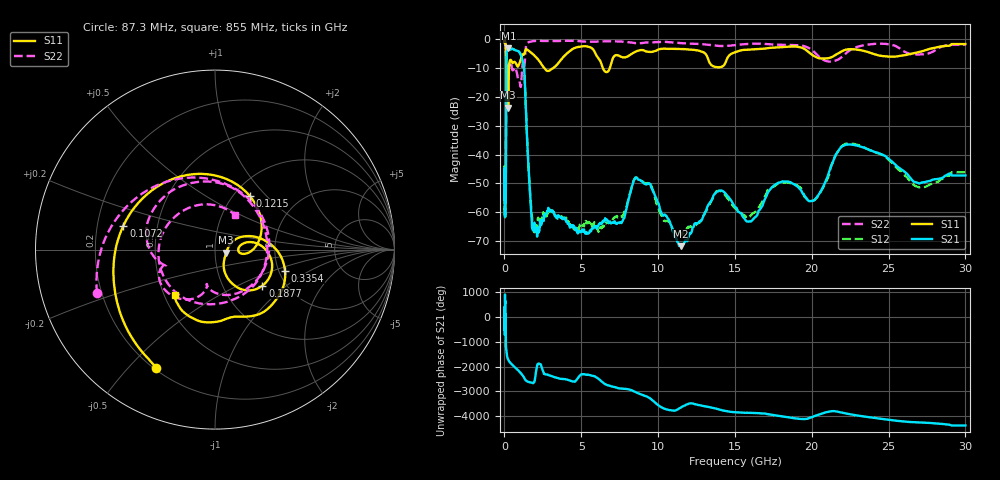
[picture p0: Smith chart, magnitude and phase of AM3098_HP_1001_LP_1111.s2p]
! Date/Time: Thu, Feb 28, 2019 8:41 AM
! Network Analyzer: Agilent Technologies E8364B Rev: A.07.50.67
! Sweep from 0.010 to 30.000 GHz, 1601 Points, Sweep Type: LOG
! Power Supply: 5.023 V, 0.002 A
# Hz S DB R 50
!freq MagS11 AngS11 MagS21 AngS21 MagS12 AngS12 MagS22 AngS22
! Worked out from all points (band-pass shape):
!   1601 points, 10 MHz to 30 GHz, reference 50 ohm
!   highest |S21| = -3.13 dB at 253.4 MHz (marker M1); lowest = -71.9 dB at 11.48 GHz (marker M2)
!   |S21| within 3 dB of the highest: 130.1 MHz to 1.112 GHz (982.2 MHz wide, 158 % of centre)
!   lowest |S11| = -23.8 dB at 239.9 MHz (marker M3), VSWR 1.14, Z = 56.6 - j1.99 ohm
!   |S11| at or under -10 dB: 192.8 MHz to 298.6 MHz (105.8 MHz wide, 43 % of centre); 2.601 GHz to 3.163 GHz (562.2 MHz wide, 19.5 % of centre); 6.406 GHz to 6.853 GHz (447.6 MHz wide, 6.75 % of centre)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
!   |S22| runs from -16.5 to -0.5 dB; largest |S21 - S12| = 0.011
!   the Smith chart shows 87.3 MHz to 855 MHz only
!   S11 on the Smith chart (normalised r, x): 87.3 MHz: 0.21, -0.60; 107.2 MHz: 0.31, +0.12; 121.5 MHz: 1.19, +0.81; 187.7 MHz: 1.53, -0.69; 335.4 MHz: 2.16, -0.61; 855 MHz: 0.57, -0.32
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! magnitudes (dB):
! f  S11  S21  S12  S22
! 10 MHz  -0.4  -45.0  -44.4  -0.6
! 38.04 MHz  -0.5  -59.9  -58.6  -1.0
! 87.3 MHz  -2.7  -54.2  -53.2  -3.1
! 107.2 MHz  -5.6  -26.9  -26.9  -7.2
! 121.5 MHz  -9.0  -10.0  -10.0  -10.8
! 144.7 MHz  -17.4  -4.4  -4.4  -13.6
! 187.7 MHz  -9.6  -3.6  -3.6  -8.9
! 239.9 MHz  -23.8  -3.1  -3.1  -10.9
! 253.4 MHz  -19.5  -3.1  -3.1  -10.6
! 335.4 MHz  -7.8  -3.4  -3.4  -7.8
! 550.5 MHz  -8.1  -3.4  -3.3  -10.7
! 855 MHz  -9.4  -4.0  -3.9  -13.0
! 1.27 GHz  -5.3  -9.7  -9.7  -9.9
! 1.775 GHz  -4.8  -62.7  -60.8  -0.6
! 2.084 GHz  -6.3  -65.8  -65.1  -0.5
! 7.926 GHz  -6.1  -59.2  -58.5  -0.9
! 9.164 GHz  -4.1  -50.3  -50.1  -1.1
! 11.48 GHz  -3.4  -71.9  -67.6  -1.3
! 13.95 GHz  -9.7  -52.6  -52.7  -2.3
! 20.2 GHz  -5.9  -55.7  -55.7  -4.6
! 22.56 GHz  -3.4  -36.5  -36.2  -3.5
! 30 GHz  -1.6  -47.3  -46.2  -1.9
